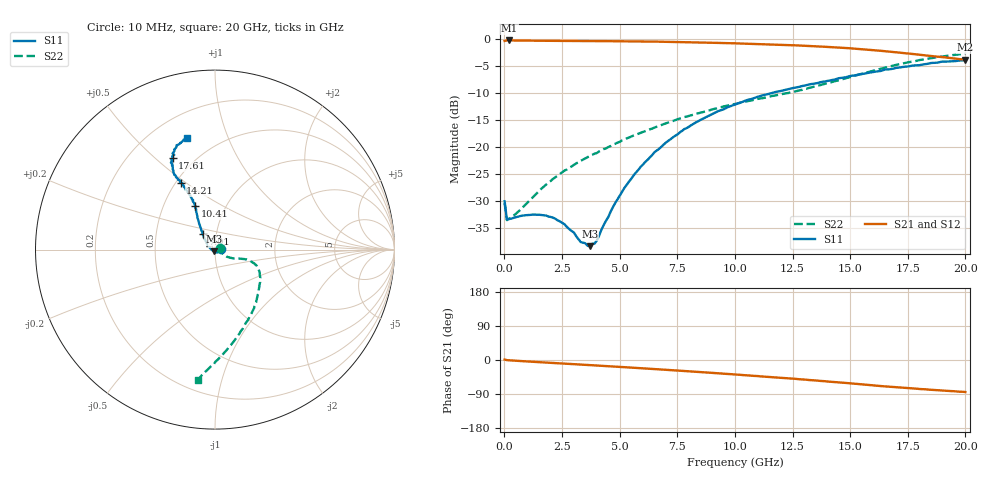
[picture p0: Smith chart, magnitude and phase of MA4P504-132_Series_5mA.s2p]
! AWR Design Environment (9226) Thu Aug 19 02:45:16 2021
! Document = '5mA'
! nPorts: 2, nXvals: 201
# GHz S DB R 50
!Freq DBS11 AngS11 DBS21 AngS21 DBS12 AngS12 DBS22 AngS22
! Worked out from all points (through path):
!   201 points, 10 MHz to 20 GHz, reference 50 ohm
!   highest |S21| = -0.24 dB at 210 MHz (marker M1); lowest = -3.8 dB at 20 GHz (marker M2)
!   group delay of S21, straight-line fit = 11.9 ps
!   lowest |S11| = -38.3 dB at 3.71 GHz (marker M3), VSWR 1.02, Z = 49.2 - j0.938 ohm
!   |S11| at or under -10 dB: start of sweep to 11.58 GHz
!   |S22| runs from -33.5 to -2.7 dB; largest |S21 - S12| = 0.03
!   S11 on the Smith chart (normalised r, x): 10 MHz: 1.06, +0.01; 7.01 GHz: 0.86, +0.15; 10.41 GHz: 0.72, +0.38; 14.21 GHz: 0.53, +0.48; 17.61 GHz: 0.38, +0.57; 20 GHz: 0.34, +0.72
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0.01  -29.99 9.0  -0.32 1.3  -0.29 0.6  -30.35 19.5
0.11  -33.35 -2.3  -0.24 -0.4  -0.23 -0.4  -33.48 -3.2
0.21  -33.28 -1.8  -0.24 -0.8  -0.23 -0.8  -33.21 -2.8
1.21  -32.47 -17.5  -0.28 -4.7  -0.27 -4.6  -29.34 -19.3
2.11  -33.03 -39.9  -0.31 -7.8  -0.30 -7.6  -25.85 -28.6
2.61  -34.26 -56.5  -0.32 -9.6  -0.32 -9.3  -24.31 -30.8
3.41  -37.66 -98.5  -0.34 -12.4  -0.33 -12.0  -22.29 -30.5
3.71  -38.30 -128.4  -0.35 -13.5  -0.34 -13.0  -21.58 -29.9
4.01  -37.27 -153.9  -0.35 -14.6  -0.35 -14.1  -21.07 -29.0
5.21  -27.50 151.0  -0.39 -19.0  -0.38 -18.3  -18.57 -24.8
5.91  -23.63 138.8  -0.42 -21.6  -0.42 -20.9  -17.32 -21.1
6.71  -20.29 130.7  -0.46 -24.7  -0.45 -24.0  -16.06 -19.0
7.01  -19.13 128.5  -0.48 -25.9  -0.48 -25.1  -15.57 -18.4
8.31  -15.39 121.3  -0.59 -31.1  -0.59 -30.1  -13.83 -17.7
10.01  -12.10 115.1  -0.77 -38.3  -0.76 -36.8  -12.00 -21.4
10.41  -11.46 114.3  -0.82 -40.1  -0.80 -38.5  -11.62 -23.3
13.41  -8.25 116.3  -1.29 -53.5  -1.20 -52.0  -8.81 -50.0
14.21  -7.56 117.3  -1.49 -57.5  -1.36 -55.9  -7.93 -58.5
16.71  -5.58 116.9  -2.31 -70.5  -2.19 -69.1  -5.06 -82.9
17.61  -4.98 114.8  -2.69 -74.7  -2.60 -73.8  -4.21 -88.8
19.01  -4.16 110.3  -3.31 -80.4  -3.34 -80.2  -3.20 -95.3
20  -3.88 104.1  -3.82 -84.6  -3.93 -84.0  -2.67 -97.5
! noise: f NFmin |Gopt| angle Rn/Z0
0.01  0  1  0  2e-20
2.21  0  1  0  2e-20
4.41  0  1  0  2e-20
6.61  0  1  0  2e-20
8.81  0  1  0  2e-20
11.11  0  1  0  2e-20
13.31  0  1  0  2e-20
15.51  0  1  0  2e-20
17.71  0  1  0  2e-20
20  0  1  0  2e-20
